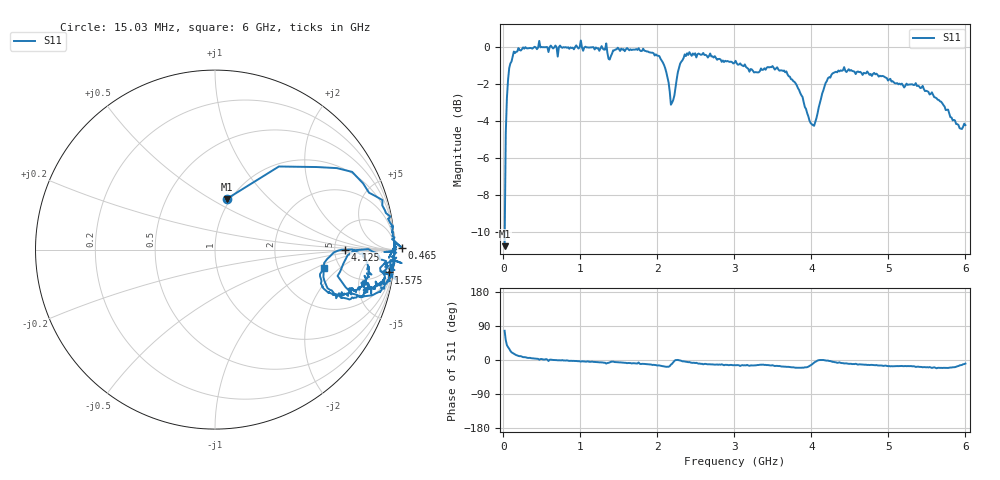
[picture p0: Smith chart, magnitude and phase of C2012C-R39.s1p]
!	Network	Analyzer	HP8753E.07.74:	Oct	30	2002	Serial	No.	JP38451487
!	Hewlett-Packard
!	7	Sep	2009	12:25:46
!	Frequency	S11
#	HZ	S	RI	R	50
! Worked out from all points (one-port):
!   400 points, 15.03 MHz to 6 GHz, reference 50 ohm
!   lowest |S11| = -10.8 dB at 15.03 MHz (marker M1), VSWR 1.81, Z = 48 + j29.6 ohm
!   |S11| at or under -10 dB: start of sweep to 16.93 MHz
!   S11 on the Smith chart (normalised r, x): 15.03 MHz: 0.96, +0.59; 465 MHz: -47, +13; 1.575 GHz: 3, -15; 4.125 GHz: 6.30, -0.04; 6 GHz: 3.77, -1.23
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1.502992e7  0.0647 0.282
3.002985e7  0.356 0.463
6.00297e7  0.679 0.454
1.350293e8  0.933 0.276
4.650277e8  1.04 0.0112
6.750266e8  1.01 0.00238
7.050265e8  0.943 -0.0135
7.650262e8  0.996 -0.00583
1.335023e9  1.01 -0.167
1.365023e9  0.922 -0.121
1.515022e9  0.971 -0.108
1.575022e9  0.967 -0.127
1.95002e9  0.939 -0.212
2.115019e9  0.814 -0.264
2.175019e9  0.683 -0.147
2.265019e9  0.855 0.00259
2.415018e9  0.965 -0.0903
2.595017e9  0.945 -0.192
3.015015e9  0.892 -0.219
3.375013e9  0.849 -0.185
3.765011e9  0.764 -0.266
3.99001e9  0.604 -0.153
4.125009e9  0.726 -0.00134
4.275009e9  0.846 -0.0719
4.515007e9  0.854 -0.151
5.265004e9  0.761 -0.22
5.625002e9  0.675 -0.271
6e9  0.607 -0.101
